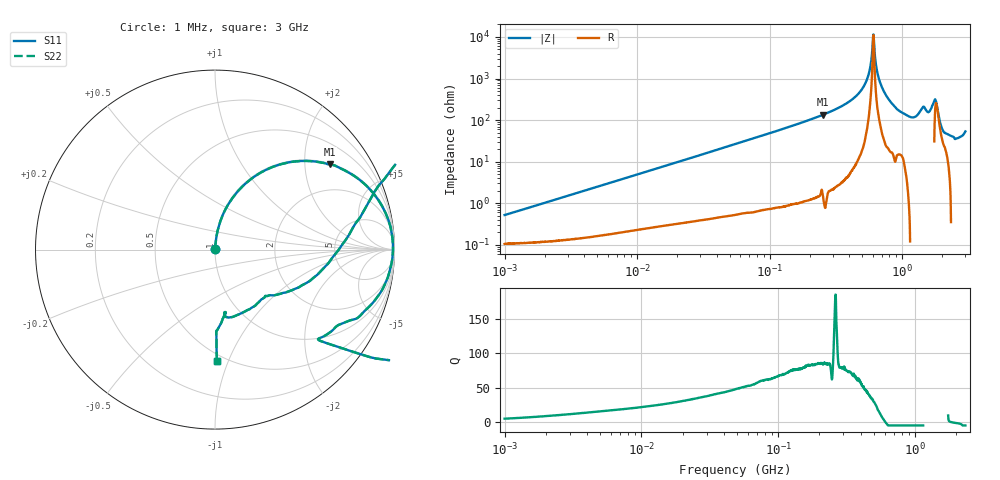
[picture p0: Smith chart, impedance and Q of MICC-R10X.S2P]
!s-Parameter Generated by FASTRON Sdn. Bhd.
!FASTRON P/N : MICC-R10X
!Keysight Technologies,E4991B,MY54100416,A.01.15
!Date: Wed Aug 26 14:49:25 2026
!Version  : Rev00 Wed Aug 26 14:49:25 2026
!Data & Calibration Information:
!PortZ  Port1:50+j0  Port2:50+j0
!When reading, reference impedance value at option line is always used.
!Remarks : This data is being provided solely for informational purposes.
!Freq	S11	S21	S12	S22
# Hz S dB R 50
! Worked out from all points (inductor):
!   1601 points, 1 MHz to 3 GHz, reference 50 ohm
!   read as one part in series: L = 80.5 nH near 1.041 MHz
!   highest Q = 87.4 at 253.3 MHz (marker M1), where L = 84.3 nH
!   self-resonance near 604.9 MHz
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1000000  -45.72 78.1  -0.01 -0.3  -0.01 -0.3  -45.72 78.1
3804036  -34.43 84.6  -0.01 -1.1  -0.01 -1.1  -34.43 84.6
1.447069e7  -23.11 83.8  -0.04 -4.0  -0.04 -4.0  -23.11 83.8
5.477226e7  -11.95 74.2  -0.33 -14.6  -0.33 -14.6  -11.95 74.2
2.083556e8  -2.81 43.0  -3.33 -46.4  -3.33 -46.4  -2.81 43.0
2.532562e8  -1.96 36.5  -4.51 -52.9  -4.51 -52.9  -1.96 36.5
4.805402e8  -0.24 11.8  -13.81 -76.6  -13.81 -76.6  -0.24 11.8
5.473095e8  -0.10 5.5  -20.32 -80.5  -20.32 -80.5  -0.10 5.5
6.049187e8  -0.07 0.2  -41.16 -18.0  -41.16 -18.0  -0.07 0.2
6.787043e8  -0.16 -6.7  -18.58 77.5  -18.58 77.5  -0.16 -6.7
7.925923e8  -0.58 -17.3  -10.50 69.1  -10.50 69.1  -0.58 -17.3
1.294266e9  -1.67 -39.6  -3.88 55.3  -3.88 55.3  -1.67 -39.6
1.388188e9  0.70 -34.1  -4.21 80.4  -4.21 80.4  0.70 -34.1
1.452135e9  3.55 -23.7  -2.93 122.0  -2.93 122.0  3.55 -23.7
1.511446e9  7.29 -5.9  2.44 169.6  2.44 169.6  7.29 -5.9
1.54974e9  8.48 10.0  4.50 -164.1  4.50 -164.1  8.48 10.0
1.629261e9  5.17 27.7  0.32 -125.8  0.32 -125.8  5.17 27.7
1.695807e9  1.24 25.9  -5.92 -94.2  -5.92 -94.2  1.24 25.9
1.773925e9  -1.65 12.4  -11.63 -42.9  -11.63 -42.9  -1.65 12.4
1.941122e9  -6.09 -26.2  -4.49 21.5  -4.49 21.5  -6.09 -26.2
2.568929e9  -8.78 -80.9  0.08 20.9  0.08 20.9  -8.78 -80.9
3e9  -4.10 -89.2  1.37 32.2  1.37 32.2  -4.10 -89.2
